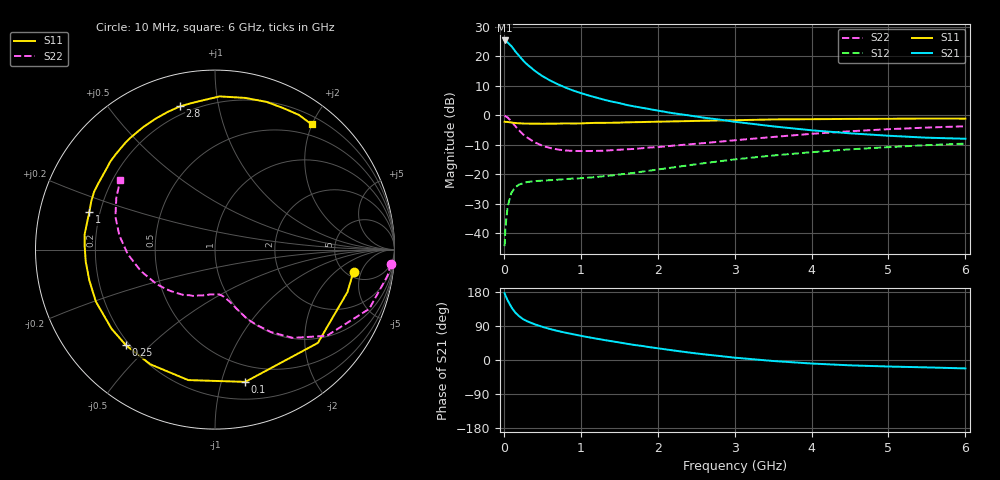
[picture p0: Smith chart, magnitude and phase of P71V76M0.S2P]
! SIEMENS Small Signal Semiconductors
! BFP196
! Si NPN RF Bipolar Junction Transistor in SOT143
! VCE = 1.75 V  IC = 6 mA
! Common Emitter S-Parameters:  May  1996
# GHz  S  MA  R  50
!  f  S11  S21  S12  S22
! GHz  MAG  ANG  MAG  ANG  MAG  ANG  MAG  ANG
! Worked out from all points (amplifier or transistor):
!   36 points, 10 MHz to 6 GHz, reference 50 ohm
!   highest |S21| = 25.4 dB at 10 MHz (marker M1)
!   |S21| within 3 dB of that: start of sweep to 129.2 MHz
!   unconditionally stable (mu >= 1): 1.022 GHz to 3.309 GHz; 5.747 GHz to end of sweep
!   at 250 MHz: K = 0.29, MSG = 20.8 dB, |S12| = -23.0 dB
!   at 1.4 GHz: K = 1.17, MAG = 10.0 dB, |S12| = -20.4 dB
!   at 6 GHz: K = 1.01, MAG = 0.2 dB, |S12| = -9.6 dB
!   S11 on the Smith chart (normalised r, x): 10 MHz: 5.81, -3.65; 100 MHz: 0.35, -1.19; 250 MHz: 0.19, -0.42; 1 GHz: 0.16, +0.14; 2.8 GHz: 0.16, +0.77; 6 GHz: 0.32, +2.00
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0.01  0.7815 -9.0  18.56 176.2  0.0061 86.8  0.9835 -4.6
0.02  0.7749 -17.8  18.12 170.3  0.0123 81.7  0.9719 -8.7
0.05  0.7739 -42.2  17.17 157.2  0.0291 69.1  0.9206 -21.0
0.1  0.756 -77.1  14.8 138.8  0.0492 53.8  0.7869 -37.6
0.15  0.7422 -101.6  12.08 124.9  0.0608 43.4  0.6557 -48.6
0.2  0.7336 -119.4  10.14 115.4  0.0676 36.4  0.556 -55.8
0.25  0.728 -132.9  8.532 107.8  0.0708 31.6  0.4775 -61.3
0.3  0.7258 -142.5  7.349 102.5  0.0742 28.9  0.4241 -65.2
0.4  0.7243 -156.4  5.716 94.3  0.0769 25.4  0.3503 -70.0
0.5  0.7209 -166.1  4.629 87.6  0.0786 24.2  0.3068 -73.6
0.6  0.7233 -174.5  3.91 81.8  0.0799 23.9  0.2805 -77.1
0.7  0.7259 178.9  3.374 76.6  0.0814 24.2  0.2646 -80.0
0.8  0.7314 173.4  2.962 72.2  0.0834 24.9  0.2546 -82.9
1  0.7307 163.3  2.385 63.9  0.0861 27.1  0.2487 -88.0
1.1  0.7401 158.7  2.18 60.1  0.0882 28.7  0.2493 -91.2
1.6  0.7625 139.8  1.499 42.8  0.103 35.3  0.2665 -106.6
2.2  0.7907 120.6  1.088 25.3  0.1313 38.9  0.3071 -124.5
2.8  0.8215 103.7  0.849 10.7  0.1669 37.6  0.358 -143.7
3.5  0.854 88.3  0.652 -2.6  0.2093 31.7  0.431 -164.1
4.5  0.8717 70.8  0.497 -14.1  0.2662 20.7  0.5383 171.7
5.5  0.8841 58.0  0.419 -19.5  0.3131 8.5  0.6216 152.2
6  0.8812 52.3  0.402 -22.2  0.3326 2.0  0.6547 143.7
